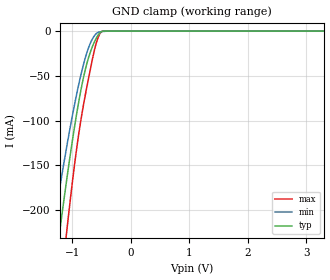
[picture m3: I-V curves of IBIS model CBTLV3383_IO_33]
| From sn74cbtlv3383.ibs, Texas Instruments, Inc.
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[Model]   CBTLV3383_IO_33
Model_type  Terminator
| variable   typ   min   max
C_comp   9.16pF   7.61pF   10.33pF
| C_tri-state   9.16pF   7.61pF   10.33pF
[Temperature Range]   40   100   -40
| Ambient temperature   25   85   -40
[Voltage range]   3.3   3   3.6
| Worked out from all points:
|   GND clamp passes 1 mA (typ) near -0.51 V on its own axis
[GND Clamp]
| CBTLV3383_IO_33
|   Voltage   I(typ)   I(min)   I(max)
-3.3V     -1.491A    -1.194A    -1.917A
-1.33V    -284.3mA   -223.7mA   -375.5mA
-1.225V   -230.2mA   -180.5mA   -306.3mA
-1.195V   -215.2mA   -168.5mA   -287.1mA
-1.09V    -164.6mA   -128.1mA   -222.3mA
-935mV    -97.21mA   -74.24mA   -137.2mA
-805mV    -51.52mA   -36.99mA   -82.01mA
-675mV    -20.93mA   -11.49mA   -38.2mA
-610mV    -10.8mA    -4.394mA   -18.8mA
-560mV    -4.932mA   -1.542mA   -7.884mA
-475mV    -100.2uA   -453.8uA   -60.55uA
3.3V      1.472nA    63.78nA    25.28pA
